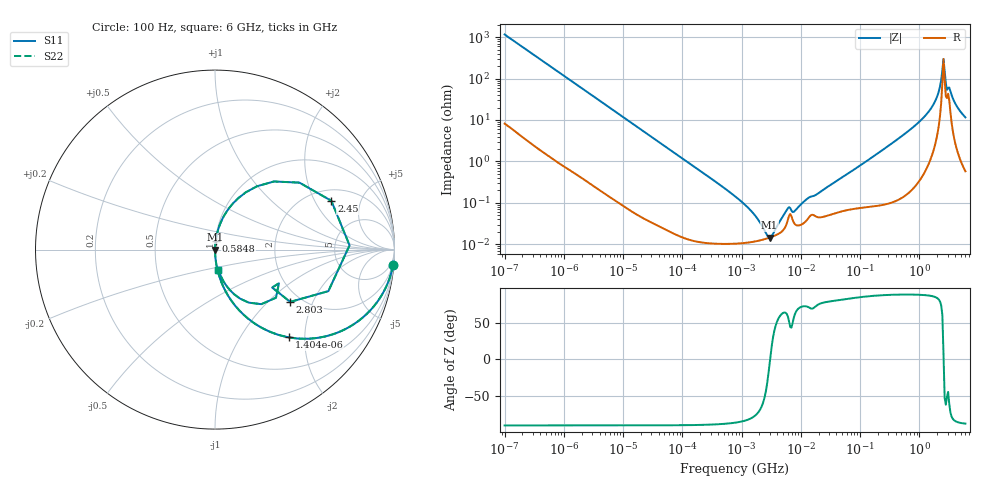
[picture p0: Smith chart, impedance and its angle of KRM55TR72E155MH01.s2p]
!Murata Part Number: KRM55TR72E155MH01
!These Parameters are Measured in Series Mode Connection
!Data Generated on Jan 08, 2026
!  o--ll--o
!Port1  Port2
!  o------o
!Operation Temp=25[degC], DC Bias Voltage=0[V]
!Freq. Start=100[Hz] Stop=6[GHz] 401[Steps]
# Hz S RI R 50
!Freq.(Hz) S11(Real) S11(Imag) S21(Real) S21(Imag) S12(Real) S12(Imag) S22(Real) S22(Imag)
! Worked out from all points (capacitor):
!   401 points, 100 Hz to 6 GHz, reference 50 ohm
!   read as one part in series: C = 1.36 uF near 109 Hz
!   lowest |Z| = 14.6 mohm at 2.968 MHz (marker M1)
!   series resonance near 3.028 MHz, so ESL is about 2 nH
!   S11 on the Smith chart (normalised r, x): 100 Hz: 1, -23; 1.404 kHz: 1.01, -1.68; 584.8 MHz: 1.00, +0.10; 2.45 GHz: 2.56, +2.75; 2.803 GHz: 1.75, -1.38; 6 GHz: 1.01, -0.23
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100  0.9921 -0.0852  0.00792 0.0852  0.00792 0.0852  0.9921 -0.0852
438  0.8756 -0.3268  0.1244 0.3268  0.1244 0.3268  0.8756 -0.3268
1404  0.4132 -0.4891  0.5868 0.4891  0.5868 0.4891  0.4132 -0.4891
2008  0.2575 -0.4339  0.7425 0.4339  0.7425 0.4339  0.2575 -0.4339
5378  0.0475 -0.2093  0.9525 0.2093  0.9525 0.2093  0.0475 -0.2093
40335  0.00115 -0.0295  0.9989 0.0295  0.9989 0.0295  0.00115 -0.0295
774597  0.000106 -0.00144  0.9999 0.00144  0.9999 0.00144  0.000106 -0.00144
1585629  0.000116 -0.000543  0.9999 0.000543  0.9999 0.000543  0.000116 -0.000543
2967816  0.000145 -1.55e-05  0.9999 1.55e-05  0.9999 1.55e-05  0.000145 -1.55e-05
6075234  0.000398 0.000634  0.9996 -0.000634  0.9996 -0.000634  0.000398 0.000634
7947587  0.000307 0.000566  0.9997 -0.000566  0.9997 -0.000566  0.000307 0.000566
1.555665e7  0.000519 0.00135  0.9995 -0.00135  0.9995 -0.00135  0.000519 0.00135
3.124326e8  0.00158 0.0247  0.9984 -0.0247  0.9984 -0.0247  0.00158 0.0247
5.847788e8  0.00379 0.0476  0.9962 -0.0476  0.9962 -0.0476  0.00379 0.0476
1.197065e9  0.0184 0.1145  0.9816 -0.1145  0.9816 -0.1145  0.0184 0.1145
1.791126e9  0.08 0.233  0.92 -0.233  0.92 -0.233  0.08 0.233
2.240541e9  0.3286 0.3795  0.6714 -0.3795  0.6714 -0.3795  0.3286 0.3795
2.450438e9  0.6482 0.272  0.3518 -0.272  0.3518 -0.272  0.6482 0.272
2.802721e9  0.4192 -0.2913  0.5808 0.2913  0.5808 0.2913  0.4192 -0.2913
3.065283e9  0.3561 -0.1876  0.6439 0.1876  0.6439 0.1876  0.3561 -0.1876
3.8344e9  0.1073 -0.2493  0.8927 0.2493  0.8927 0.2493  0.1073 -0.2493
6e9  0.0188 -0.1131  0.9812 0.1131  0.9812 0.1131  0.0188 -0.1131
